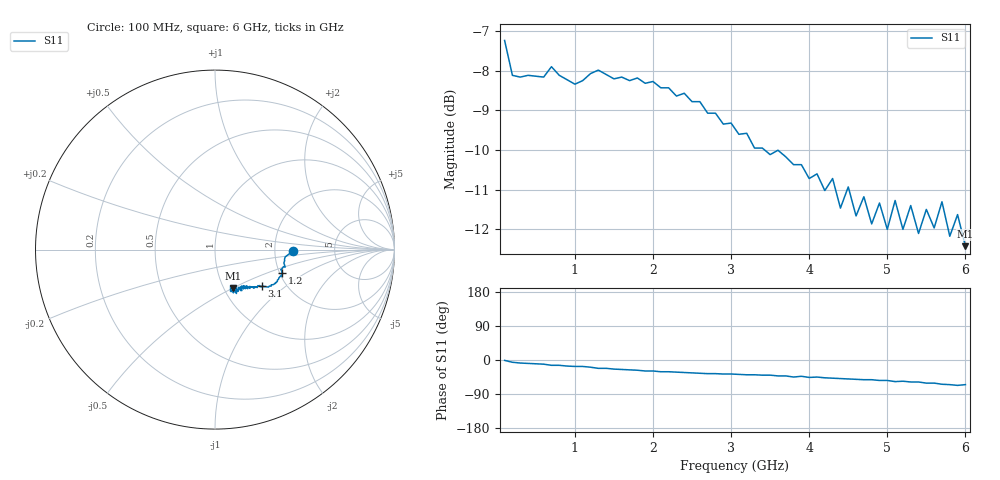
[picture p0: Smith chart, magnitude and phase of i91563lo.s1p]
!  IAM-91563  Typical Reflection Coefficients, LO port
!  Tc=25 C, Vdd= 3 V
!  LAST UPDATED 02-25-97
# ghz s ma r 50
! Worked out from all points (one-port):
!   60 points, 100 MHz to 6 GHz, reference 50 ohm
!   lowest |S11| = -12.4 dB at 6 GHz (marker M1), VSWR 1.63, Z = 55.1 - j25.3 ohm
!   |S11| at or under -10 dB: 3.429 GHz to end of sweep
!   S11 on the Smith chart (normalised r, x): 100 MHz: 2.54, -0.05; 1.2 GHz: 2.06, -0.63; 3.1 GHz: 1.51, -0.69; 6 GHz: 1.10, -0.51
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0.1  0.435 -1.0
0.2  0.393 -6.0
0.7  0.403 -14.0
0.9  0.388 -16.0
1.2  0.395 -19.0
1.6  0.391 -25.0
2.4  0.373 -33.0
3.1  0.331 -38.0
3.8  0.303 -45.0
4.2  0.281 -47.0
4.3  0.291 -48.0
4.4  0.267 -49.0
4.5  0.284 -50.0
4.6  0.261 -51.0
4.7  0.276 -52.0
4.8  0.255 -52.0
4.9  0.271 -54.0
5  0.251 -54.0
5.1  0.273 -57.0
5.2  0.251 -56.0
5.3  0.269 -58.0
5.4  0.248 -58.0
5.5  0.266 -61.0
5.6  0.252 -61.0
5.7  0.272 -64.0
5.8  0.246 -65.0
5.9  0.262 -67.0
6  0.239 -65.0
